(* Logix 5000 AddOnInstructionDefinition export; software revision 16.04 *)

ADD_ON_INSTRUCTION AMCI_ANG1E_Home_CCW   (* revision 1.1, vendor AMCI *)
// Revision note:
// Version 1.1 added the slot_axis number and the input parameters can now be tags or discrete values.
VAR_INPUT
   slot_axis_number : INT; {required}
   Programmed_Speed : DINT; {required}
   Acceleration : INT; {required}
   Deceleration : INT; {required}
END_VAR
VAR_IN_OUT
   AMCI_ANG1E_output_data : INT[10]; {required}
END_VAR
VAR
   Upper_Result_X_1000 : DINT;
   command_data_block : INT[10];
        [0]   // Command Bits MSW
        [1]   // Command Bits LSW
        [2]   // Upper Target Position
        [3]   // Lower Target Position
        [4]   // Upper Programmed Speed
        [5]   // Lower Programmed Speed
   index : INT;
END_VAR

ROUTINE Logic   (* ladder *)
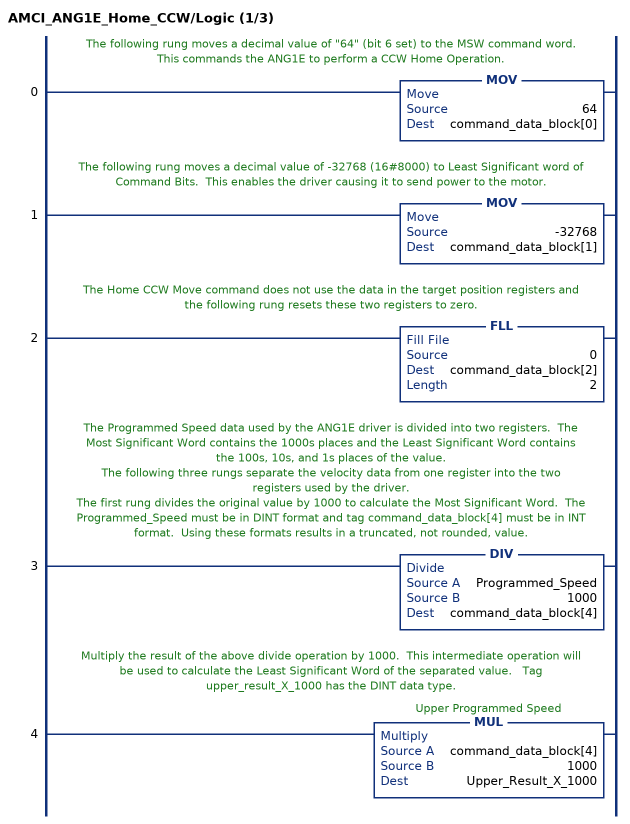
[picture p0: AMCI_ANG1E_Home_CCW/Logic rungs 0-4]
   // The following rung moves a decimal value of "64" (bit 6 set) to the MSW command word.  This commands the ANG1E to perform a CCW Home Operation.
   0: MOV(64,command_data_block[0]);
   // The following rung moves a decimal value of -32768 (16#8000) to Least Significant word of Command Bits.  This enables the driver causing it to send power to the motor.
   1: MOV(-32768,command_data_block[1]);
   // The Home CCW Move command does not use the data in the target position registers and the following rung resets these two registers to zero.
   2: FLL(0,command_data_block[2],2);
   // The Programmed Speed data used by the ANG1E driver is divided into two registers.  The Most Significant Word contains the 1000s places and the Least Significant Word contains the 100s, 10s, and 1s places of the value.
   // The following three rungs separate the velocity data from one register into the two registers used by the driver.
   // The first rung divides the original value by 1000 to calculate the Most Significant Word.  The Programmed_Speed must be in DINT format and tag command_data_block[4] must be in INT format.  Using these formats results in a truncated, not rounded, value.
   3: DIV(Programmed_Speed,1000,command_data_block[4]);
   // Multiply the result of the above divide operation by 1000.  This intermediate operation will be used to calculate the Least Significant Word of the separated value.   Tag upper_result_X_1000 has the DINT data type.
   4: MUL(command_data_block[4],1000,Upper_Result_X_1000);
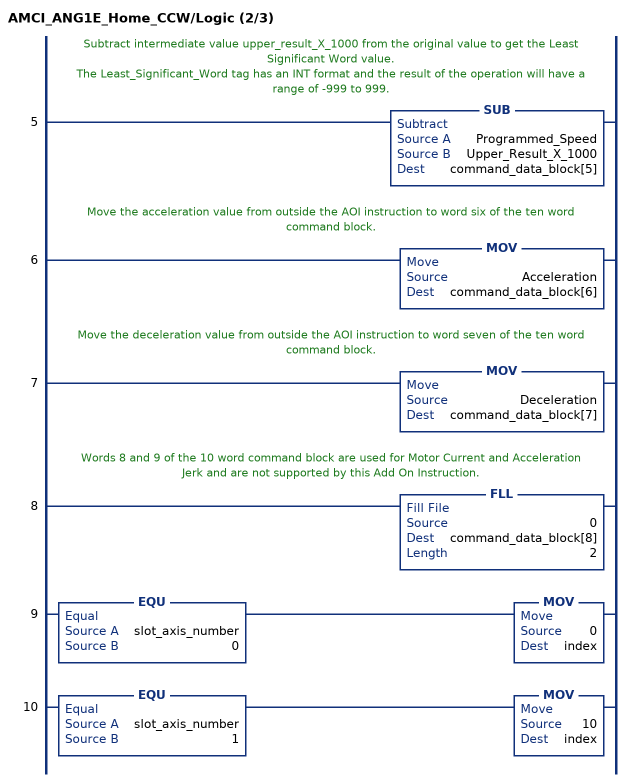
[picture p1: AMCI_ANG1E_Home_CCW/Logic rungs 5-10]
   // Subtract intermediate value upper_result_X_1000 from the original value to get the Least Significant Word value.
   // The Least_Significant_Word tag has an INT format and the result of the operation will have a range of -999 to 999.
   5: SUB(Programmed_Speed,Upper_Result_X_1000,command_data_block[5]);
   // Move the acceleration value from outside the AOI instruction to word six of the ten word command block.
   6: MOV(Acceleration,command_data_block[6]);
   // Move the deceleration value from outside the AOI instruction to word seven of the ten word command block.
   7: MOV(Deceleration,command_data_block[7]);
   // Words 8 and 9 of the 10 word command block are used for Motor Current and Acceleration Jerk and are not supported by this Add On Instruction.
   8: FLL(0,command_data_block[8],2);
   9: EQU(slot_axis_number,0)MOV(0,index);
   10: EQU(slot_axis_number,1)MOV(10,index);
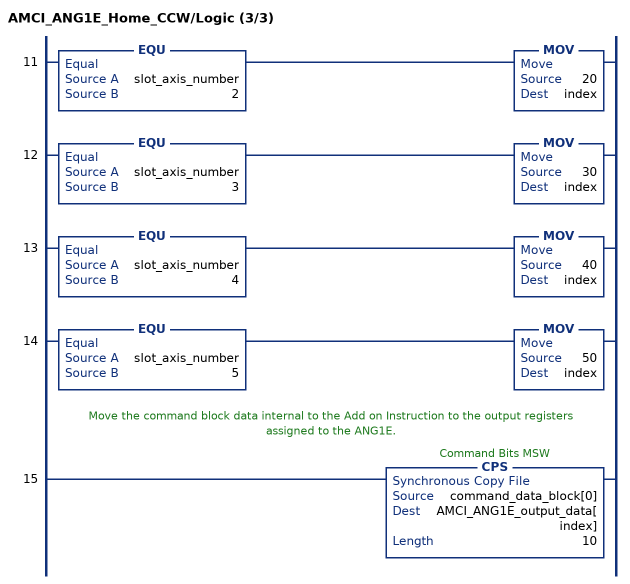
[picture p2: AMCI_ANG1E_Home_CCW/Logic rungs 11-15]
   11: EQU(slot_axis_number,2)MOV(20,index);
   12: EQU(slot_axis_number,3)MOV(30,index);
   13: EQU(slot_axis_number,4)MOV(40,index);
   14: EQU(slot_axis_number,5)MOV(50,index);
   // Move the command block data internal to the Add on Instruction to the output registers assigned to the ANG1E.
   15: CPS(command_data_block[0],AMCI_ANG1E_output_data[index],10);
END_ROUTINE
END_ADD_ON_INSTRUCTION
